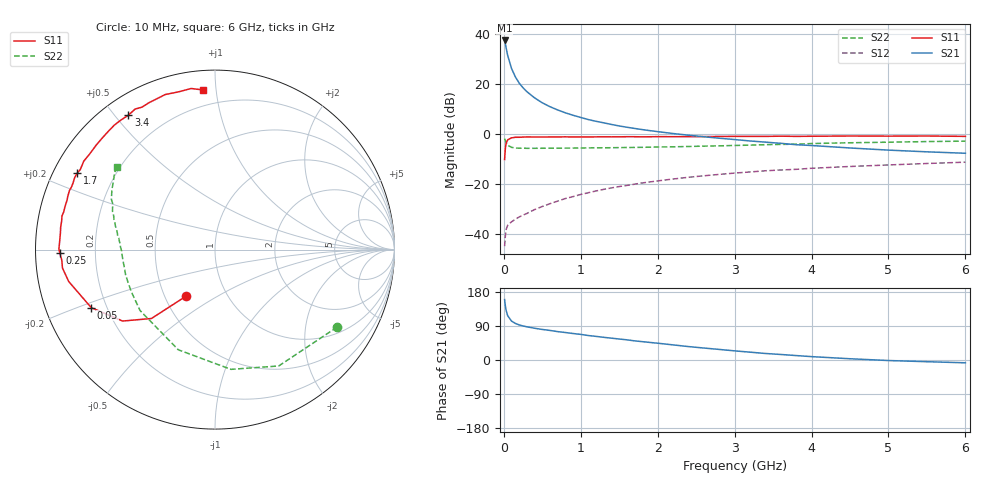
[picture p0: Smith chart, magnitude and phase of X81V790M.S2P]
! SIEMENS Small Signal Semiconductors
! BFP136W
! Si NPN RF Bipolar Junction Transistor in SOT343
! VCE = 1.75 V  IC = 90 mA
! Common Emitter S-Parameters:  September  1994
# GHz  S  MA  R  50
!  f  S11  S21  S12  S22
! GHz  MAG  ANG  MAG  ANG  MAG  ANG  MAG  ANG
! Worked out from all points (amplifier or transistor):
!   40 points, 10 MHz to 6 GHz, reference 50 ohm
!   highest |S21| = 37.4 dB at 10 MHz (marker M1)
!   |S21| within 3 dB of that: start of sweep to 30.2 MHz
!   unconditionally stable (mu >= 1): 482.2 MHz to 2.916 GHz
!   at 200 MHz: K = 0.70, MSG = 26.7 dB, |S12| = -33.2 dB
!   at 1.5 GHz: K = 1.11, MAG = 10.1 dB, |S12| = -21.1 dB
!   at 6 GHz: K = 0.99, MSG = 1.8 dB, |S12| = -11.3 dB
!   S11 on the Smith chart (normalised r, x): 10 MHz: 0.64, -0.37; 50 MHz: 0.14, -0.22; 250 MHz: 0.07, -0.01; 1.7 GHz: 0.07, +0.26; 3.4 GHz: 0.07, +0.54; 6 GHz: 0.11, +0.92
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0.01  0.3071 -122.0  73.71 159.5  0.0057 69.2  0.8059 -32.4
0.02  0.5224 -132.7  62.74 142.6  0.0092 55.7  0.7392 -61.3
0.03  0.6508 -142.3  52.37 130.7  0.0123 47.9  0.6731 -82.4
0.05  0.7617 -154.9  36.96 116.8  0.0149 38.2  0.5945 -110.1
0.1  0.8343 -167.7  20.29 102.7  0.0175 35.4  0.5381 -140.9
0.15  0.856 -173.1  13.77 96.5  0.0197 38.4  0.5219 -153.4
0.2  0.8557 -176.1  10.33 92.6  0.0219 41.0  0.5176 -160.1
0.25  0.8647 -178.7  8.336 89.8  0.0238 44.3  0.5174 -164.4
0.3  0.8698 179.8  6.969 87.6  0.0257 47.9  0.515 -167.3
0.4  0.8662 176.2  5.245 83.8  0.0307 52.0  0.5153 -171.1
0.5  0.8663 173.7  4.181 80.6  0.0354 55.1  0.5164 -173.7
0.6  0.8689 171.8  3.491 78.0  0.0403 57.5  0.5176 -175.5
0.7  0.8692 169.4  3.009 74.9  0.0454 59.6  0.5185 -176.7
0.9  0.8686 166.0  2.356 69.9  0.0558 60.8  0.5206 -179.3
1.1  0.8692 161.5  1.93 64.5  0.0668 61.2  0.5247 179.1
1.7  0.8782 151.0  1.285 50.5  0.0989 59.1  0.5369 174.2
2.2  0.8784 142.6  1.017 39.9  0.1253 55.3  0.5517 170.4
3.2  0.892 125.8  0.722 20.7  0.1734 45.7  0.5959 161.4
3.4  0.8908 122.8  0.685 17.2  0.1831 43.5  0.6091 159.6
4.5  0.9073 107.8  0.523 3.3  0.2231 33.2  0.6651 149.7
5.5  0.9074 98.4  0.438 -4.5  0.2561 25.2  0.7025 142.9
6  0.8919 94.3  0.41 -7.4  0.2722 20.8  0.7168 139.9
